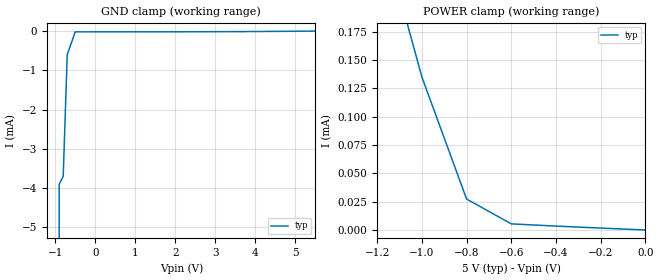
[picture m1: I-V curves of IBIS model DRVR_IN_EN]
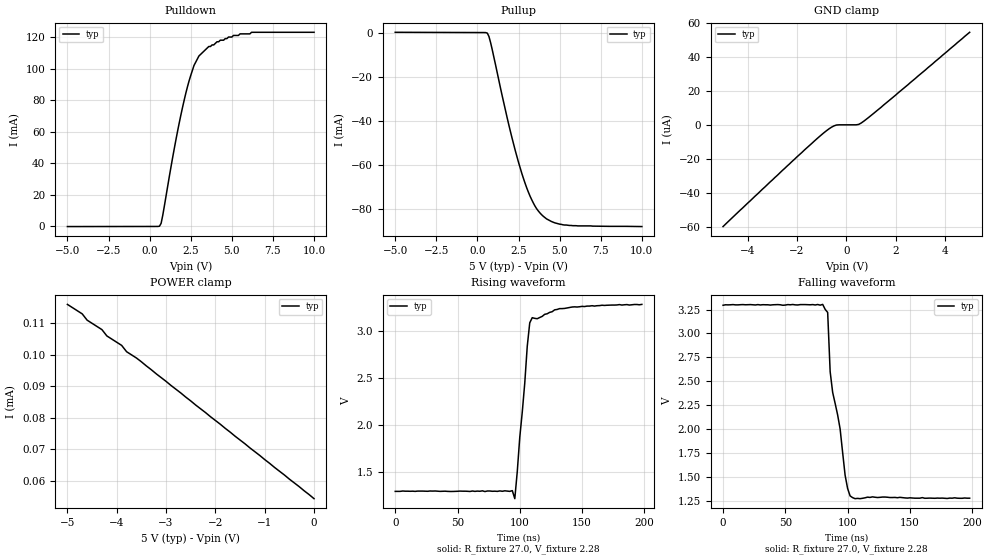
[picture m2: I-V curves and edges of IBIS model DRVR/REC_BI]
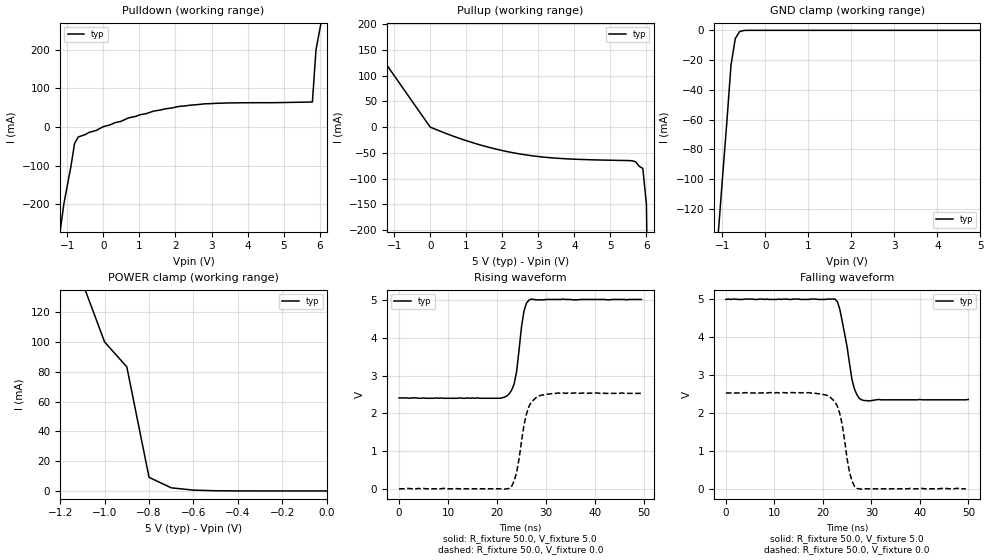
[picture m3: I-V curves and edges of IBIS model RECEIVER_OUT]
|   Texas Instruments Incorporated
|   Data Transmissions Products
|   IBIS Model for SN65HVD1787
|   SOIC 8-pin (D), PDIP 8-pin (P), VCC=5V
[IBIS Ver]   3.2
[Comment char]   |_char
[File name]   sllc357.ibs
[File Rev]   1.0
[Date]   13Aug08
[Source]   File originated at Texas Instruments Incorporated.
   Data Transmission Products Group.
[Notes]
[Disclaimer]
(C) Copyright Texas Instruments Incorporated 2002
   All rights reserved
  Texas Instruments Incorporated hereby grants the user of this IBIS
model a non-exclusive, nontransferable license to use this IBIS model
under the following terms.  Before using this IBIS model, the user
should read this license.  If the user does not accept these terms,
the IBIS model should be returned to Texas Instruments within 30 days.
  The user is granted this license only to use the IBIS model and
is not granted rights to sell, load, rent, lease or license the IBIS
model in whole or in part, or in modified form to anyone other than
user.  User may modify the IBIS model to suit its specific applications
but rights to derivative works and such modifications shall belong to
Texas Instruments.
  This IBIS model is provided on an "AS IS" basis and Texas Instruments
makes absolutely no warranty with respect to the information contained
herein.  TEXAS INSTRUMENTS DISCLAIMS AND CUSTOMER WAIVES ALL WARRANTIES,
EXPRESS OR IMPLIED, INCLUDING WARRANTIES OF MERCHANTABILITY OR FITNESS
FOR A PARTICULAR PURPOSE. The entire risk as to quality and performance
is with the Customer. ACCORDINGLY, IN NO EVENT SHALL THE COMPANY BE LIABLE
FOR ANY DAMAGES, WHETHER IN CONTRACT OR TORT,INCLUDING ANY LOST PROFITS
OR OTHER INCIDENTAL, CONSEQUENTIAL, EXEMPLARY, OR PUNITIVE DAMAGES ARISING
OUT OF THE USE OR APPLICATION OF THE IBIS model provided in this package.
Further, Texas Instruments reserves the right to discontinue or make changes
without notice to any product herein to improve reliability, function, or
design. Texas Instruments does not convey any license under patent rights
or any other intellectual property rights, including those of third parties.
Contact Texas Instruments at ATTN:DATA TRANSMISSIONS
[Copyright]   Copyright 2002, Texas Instruments, All Rights Reserved
[Component]   HVD1787_D
[Manufacturer]  Texas Instruments Incorporated
[Package]
|   typ   min   max
R_pkg   0.1017   0.0608   0.1359
L_pkg   1.9890nH   1.6927nH   2.3143nH
C_pkg   0.3794pF   0.3519pF   0.3977pF
[Pin]   signal_name   model_name   R_pin   L_pin   C_pin
1   R   RECEIVER_OUT   0.108   1.993n   0.363p
2   REB   DRVR_IN_EN   0.103   1.929n   0.373p
3   DE   DRVR_IN_EN   0.103   1.932n   0.373p
4   D   DRVR_IN_EN   0.107   2.016n   0.352p
5   GND   GND   0.064   1.778n   0.394p
6   A   DRVR/REC_BI   0.131   2.258n   0.391p
7   B   DRVR/REC_BI   0.136   2.314n   0.391p
8   VCC   POWER   0.061   1.693n   0.398p
[Diff_pin]   inv_pin   vdiff   tdelay_typ   tdelay_min   tdelay_max
| The 'A' pin is Diff_pin and the 'B' pin is the inv_pin
6   7   0.200   0   0   0
[Component]   HVD1787_P
[Manufacturer]  Texas Instruments Incorporated
[Package]
|   typ   min   max
R_pkg   0.0833   0.0374   0.1222
L_pkg   2.7019nH   1.3887nH   3.6744nH
C_pkg   0.6414pF   0.3892pF   0.8943pF
[Pin]   signal_name   model_name   R_pin   L_pin   C_pin
1   R   RECEIVER_OUT   0.078   3.269n   0.675p
2   REB   DRVR_IN_EN   0.100   2.510n   0.648p
3   DE   DRVR_IN_EN   0.111   2.858n   0.640p
4   D   DRVR_IN_EN   0.074   2.765n   0.640p
5   GND   GND   0.037   1.389n   0.389p
6   A   DRVR/REC_BI   0.105   3.674n   0.894p
7   B   DRVR/REC_BI   0.122   2.925n   0.663p
8   VCC   POWER   0.038   2.226n   0.583p
[Diff_pin]   inv_pin   vdiff   tdelay_typ   tdelay_min   tdelay_max
| The 'A' pin is Diff_pin and the 'B' pin is the inv_pin
6   7   0.200   0   0   0
| Models and submodels in the file (3): DRVR_IN_EN (Input), DRVR/REC_BI (I/O), RECEIVER_OUT (3-state)
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|   Driver Input / Receiver Enable Model
[Model]   DRVR_IN_EN
Model_type   Input
|Signals   D,DE,RE
Vinh = 2.0
Vinl = 0.8
|   typ   min   max
C_comp   1.0pF   NA   NA
|   typ   min   max
[Temperature Range]   25.0   -40   105
[Voltage range]   5.0V   4.5V   5.5V
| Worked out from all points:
|   GND clamp passes 1 mA (typ) near -0.71 V on its own axis
|   POWER clamp passes 1 mA (typ) near -2.08 V on its own axis
[GND_clamp]
|   Voltage   I(typ)   I(min)   I(max)
-5.5V     -8.7A      NA         NA
-2V       -1.9A      NA         NA
-900mV    -3.9mA     NA         NA
-800mV    -3.7mA     NA         NA
-700mV    -600uA     NA         NA
-500mV    -16uA      NA         NA
5.5V      4.37uA     NA         NA
[Power_clamp]
| Note that the[POWER_clamp]voltage table is referenced to Vcc
| and is calculated using Vtable=Vcc - Vmeasured.
|   Voltage   I(typ)   I(min)   I(max)
-5.5V     4.1mA      NA         NA
-1.2V     279uA      NA         NA
-1V       135uA      NA         NA
-800mV    27.3uA     NA         NA
-600mV    5.38uA     NA         NA
0V        8.71nA     NA         NA
|   Driver Output / Receiver Input Model
[Model]   DRVR/REC_BI
Model_type   I/O
| Signals   A,B
Vinl = 0.9V
Vinh = 2.8V
Vmeas = 1.7V   |Reference voltage for timing measurements
Cref = 50pF   |Timing specification test load capacitance value
Rref = 54   |Note: 54 Ohm load; single-ended configuration
|   Timing specification test load voltage
| variable   typ   min   max
C_comp   1.0pF   NA   NA
|   typ   min   max
[Temperature Range]   25.0   -40   105
[Voltage range]   5.0V   4.5V   5.5V
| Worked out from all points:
|   slope of the pulldown table from 0 to 0.75 V, typ, clamps not added: 165 ohm
|   slope of the pullup table from 0 to 0.75 V, typ, clamps not added: 237 ohm
|   rising waveform, R_fixture 27.0, V_fixture 2.28: 20-80 % time 7.36ns typ, NA min, NA max; typ from 1.29 V to 3.29 V
|   falling waveform, R_fixture 27.0, V_fixture 2.28: 20-80 % time 11.6ns typ, NA min, NA max; typ from 3.29 V to 1.28 V
[Pulldown]
|   Voltage   I(typ)   I(min)  I(max)
-5V       -95.8uA    NA         NA
600mV     118uA      NA         NA
700mV     1.98mA     NA         NA
800mV     7.06mA     NA         NA
1.5V      49.3mA     NA         NA
2.1V      79.9mA     NA         NA
2.4V      92.2mA     NA         NA
2.7V      102mA      NA         NA
3V        108mA      NA         NA
4.1V      117mA      NA         NA
5.5V      122mA      NA         NA
10V       123mA      NA         NA
[Pullup]
|   Voltage   I(typ)   I(min)   I(max)
| Note that the[Pullup]voltage table is referenced to Vcc
| and is calculated using Vtable=Vcc - Vmeasured.
-5V       191uA      NA         NA
600mV     -172uA     NA         NA
700mV     -1.7mA     NA         NA
800mV     -4.46mA    NA         NA
1.9V      -41.5mA    NA         NA
2.5V      -58.8mA    NA         NA
3.1V      -72.3mA    NA         NA
3.4V      -77.2mA    NA         NA
3.7V      -80.8mA    NA         NA
4.2V      -84.4mA    NA         NA
5.2V      -87.1mA    NA         NA
10V       -87.9mA    NA         NA
[GND_clamp]
|   Voltage   I(typ)   I(min)   I(max)
| Outputs in High Impedance (off)
-5V       -59.8uA    NA         NA
-2V       -18.8uA    NA         NA
-800mV    -3.39uA    NA         NA
-600mV    -1.37uA    NA         NA
-400mV    -110nA     NA         NA
400mV     11.7nA     NA         NA
600mV     1.05uA     NA         NA
1.4V      10.2uA     NA         NA
5V        54.4uA     NA         NA
[POWER_clamp]
|   Voltage   I(typ)   I(min)   I(max)
| Note that the [POWER_clamp] voltage table is referenced to Vcc
| and is calculated using Vtable = Vcc - Vmeasured.
| Outputs in Tri-state.
-5V       116uA      NA         NA
-4.7V     113uA      NA         NA
-4.6V     111uA      NA         NA
-4.3V     108uA      NA         NA
-4.2V     106uA      NA         NA
-3.9V     103uA      NA         NA
-3.8V     101uA      NA         NA
-3.5V     97.8uA     NA         NA
0V        54.4uA     NA         NA
[Ramp]
|   typ   min   max
dV/dt_r   1.30V/7.615ns   NA   NA
dV/dt_f   1.50V/13.55ns   NA   NA
R_load = 27ohm | Note: The measurement is on a single-ended configuration
|   with 54ohm line-to-line.
[Rising Waveform]
R_fixture = 27.0
V_fixture = 2.28
C_fixture = 0p
L_fixture = 0n
|   V(typ)   V(min)  V(max)
0s        1.29V      NA         NA
94ns      1.298V     NA         NA
96ns      1.212V     NA         NA
100ns     1.869V     NA         NA
104ns     2.448V     NA         NA
106ns     2.841V     NA         NA
108ns     3.091V     NA         NA
110ns     3.146V     NA         NA
142ns     3.26V      NA         NA
198ns     3.288V     NA         NA
[Falling Waveform]
R_fixture = 27.0
V_fixture = 2.28
C_fixture = 0p
L_fixture = 0n
|   V(typ)   V(min)  V(max)
0s        3.295V     NA         NA
80ns      3.304V     NA         NA
84ns      3.22V      NA         NA
86ns      2.601V     NA         NA
88ns      2.385V     NA         NA
94ns      2.002V     NA         NA
98ns      1.519V     NA         NA
100ns     1.381V     NA         NA
102ns     1.303V     NA         NA
198ns     1.279V     NA         NA
|   Receiver Output Model
[Model]   RECEIVER_OUT
Model_type   3-state
| Signals   R
Vmeas = 2.2V   |Reference voltage for timing measurements
Cref = 15pF   |Timing specification test load capacitance value
Vref = 0   |Timing specification test load voltage; GND
| variable   typ   min   max
C_comp   1.0pF   NA   NA
|   typ   min   max
[Temperature Range]   25.0   -40   105
[Voltage range]   5.0V   4.5V   5.5V
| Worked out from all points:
|   slope of the pulldown table from 0 to 0.75 V, typ, clamps not added: 31.8 ohm
|   slope of the pullup table from 0 to 0.75 V, typ, clamps not added: 36.9 ohm
|   GND clamp passes 1 mA (typ) near -0.60 V on its own axis
|   POWER clamp passes 1 mA (typ) near -0.63 V on its own axis
|   rising waveform, R_fixture 50.0, V_fixture 5.0: 20-80 % time 1.52ns typ, NA min, NA max; typ from 2.41 V to 5.01 V
|   falling waveform, R_fixture 50.0, V_fixture 5.0: 20-80 % time 2.09ns typ, NA min, NA max; typ from 4.99 V to 2.36 V
|   rising waveform, R_fixture 50.0, V_fixture 0.0: 20-80 % time 2.01ns typ, NA min, NA max; typ from 0.01 V to 2.53 V
|   falling waveform, R_fixture 50.0, V_fixture 0.0: 20-80 % time 2.01ns typ, NA min, NA max; typ from 2.53 V to 0.01 V
[Pulldown]
|   Voltage   I(typ)   I(min)  I(max)
-5V       -2.8A      NA         NA
-2.1V     -900mA     NA         NA
-1.1V     -200mA     NA         NA
-900mV    -101mA     NA         NA
-800mV    -42.3mA    NA         NA
-700mV    -25.5mA    NA         NA
700mV     24mA       NA         NA
2.8V      60.2mA     NA         NA
5.8V      65mA       NA         NA
5.9V      200mA      NA         NA
6.1V      300mA      NA         NA
10V       12A        NA         NA
[Pullup]
|   Voltage   I(typ)   I(min)  I(max)
| Note that the[Pullup]voltage table is referenced to Vcc
| and is calculated using Vtable=Vcc - Vmeasured.
-5V       500mA      NA         NA
-2V       200mA      NA         NA
-1V       100mA      NA         NA
0V        57uA       NA         NA
1.4V      -34.8mA    NA         NA
2.6V      -53.3mA    NA         NA
3.6V      -60.7mA    NA         NA
5.7V      -67.1mA    NA         NA
5.9V      -80mA      NA         NA
6V        -150mA     NA         NA
7V        -5.5A      NA         NA
10V       -22.5A     NA         NA
[GND_clamp]
|   Voltage   I(typ)   I(min)   I(max)
| Outputs in High Impedance (off)
-5V       -1.7A      NA         NA
-2V       -480mA     NA         NA
-1V       -100mA     NA         NA
-900mV    -63.1mA    NA         NA
-800mV    -23.5mA    NA         NA
-700mV    -5.53mA    NA         NA
-600mV    -837uA     NA         NA
-400mV    -4.64uA    NA         NA
5V        91.2pA     NA         NA
[POWER_clamp]
|   Voltage   I(typ)   I(min)   I(max)
| Note that the [POWER_clamp] voltage table is referenced to Vcc
| and is calculated using Vtable = Vcc - Vmeasured.
| Outputs in Tri-state.
-5V       1.7A       NA         NA
-2V       500mA      NA         NA
-1V       100mA      NA         NA
-900mV    83.3mA     NA         NA
-800mV    9.11mA     NA         NA
-700mV    2.08mA     NA         NA
-600mV    537uA      NA         NA
-500mV    126uA      NA         NA
0V        91.2pA     NA         NA
[Ramp]
|   typ   min   max
dV/dt_r   1.70V/1834ps   NA   NA
dV/dt_f   1.70V/2067ps   NA   NA
R_load = 50
[Rising Waveform]
R_fixture = 50.0
V_fixture = 5.0
V_fixture_min = 4.5
V_fixture_max = 5.5
C_fixture = 0p
L_fixture = 0n
|   V(typ)   V(min)  V(max)
0s        2.41V      NA         NA
20.5ns    2.4V       NA         NA
22ns      2.46V      NA         NA
23.5ns    2.78V      NA         NA
24ns      3.11V      NA         NA
25ns      4.29V      NA         NA
25.5ns    4.7V       NA         NA
26ns      4.91V      NA         NA
27ns      5.02V      NA         NA
49.5ns    5.01V      NA         NA
[Falling Waveform]
R_fixture = 50.0
V_fixture = 5.0
V_fixture_min = 4.5
V_fixture_max = 5.5
C_fixture = 0p
L_fixture = 0n
|   V(typ)   V(min)  V(max)
0s        4.99V      NA         NA
22.5ns    5V         NA         NA
23ns      4.93V      NA         NA
23.5ns    4.73V      NA         NA
25ns      3.74V      NA         NA
26ns      2.89V      NA         NA
26.5ns    2.64V      NA         NA
27.5ns    2.39V      NA         NA
29.5ns    2.32V      NA         NA
50ns      2.36V      NA         NA
[Rising Waveform]
R_fixture = 50.0
V_fixture = 0.0
C_fixture = 0p
L_fixture = 0n
|   V(typ)   V(min)  V(max)
0s        10mV       NA         NA
22.5ns    20mV       NA         NA
23ns      80mV       NA         NA
24ns      440mV      NA         NA
25.5ns    1.69V      NA         NA
26ns      1.98V      NA         NA
27ns      2.3V       NA         NA
28ns      2.42V      NA         NA
32.5ns    2.54V      NA         NA
49.5ns    2.53V      NA         NA
[Falling Waveform]
R_fixture = 50.0
V_fixture = 0.0
C_fixture = 0p
L_fixture = 0n
|   V(typ)   V(min)  V(max)
0s        2.53V      NA         NA
17ns      2.54V      NA         NA
21.5ns    2.42V      NA         NA
22.5ns    2.3V       NA         NA
23.5ns    1.98V      NA         NA
24ns      1.69V      NA         NA
25.5ns    440mV      NA         NA
26.5ns    80mV       NA         NA
27ns      20mV       NA         NA
49.5ns    10mV       NA         NA
